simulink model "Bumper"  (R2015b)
settings: Solver=VariableStepAuto  StartTime=0.0  StopTime=10.0  RelTol=1e-3
libraries: vexarmcortexlib x5

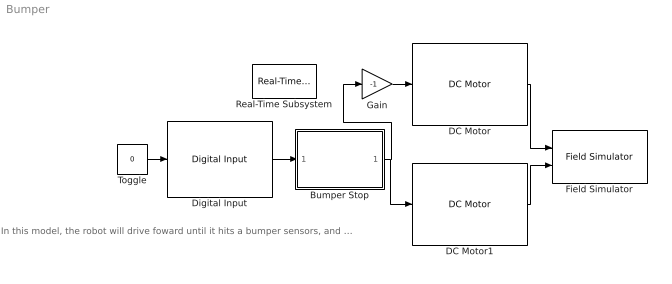
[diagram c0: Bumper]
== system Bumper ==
  note: In this model, the robot will drive foward until it hits a bumper sensors, and then will stop.
  Bumper Stop : Stateflow chart  TreatAsAtomicUnit=on
  DC Motor : vexarmcortexlib/DC Motor  motor=3  scaleFactor=1/13.5  SimulationOut=on
  DC Motor1 : vexarmcortexlib/DC Motor  motor=7  scaleFactor=1/13.5  SimulationOut=on
  Digital Input : vexarmcortexlib/Digital Input  inChan=1  SimulationIn=on
  Field Simulator : vexarmcortexlib/Utilities/Field Simulator  radius=2.5  space=10  range=200
  Gain : Gain  Gain=-1
  Real-Time Subsystem : vexarmcortexlib/Utilities/Real-Time Subsystem  x=1
  Toggle : Constant  Value=0
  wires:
  DC Motor/1 -> Field Simulator/1
  DC Motor1/1 -> Field Simulator/2
  Gain/1 -> DC Motor/1
  Digital Input/1 -> Bumper Stop/1(bumper)
  Bumper Stop/1(speed) -> DC Motor1/1, Gain/1
  Toggle/1 -> Digital Input/1

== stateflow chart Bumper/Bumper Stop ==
  state Drive_Forward
    during:
    speed = 100;
  state Stop
    during:
    speed = 0;
  (default) -> Drive_Forward : {speed = 0;}
  Drive_Forward -> Stop : [bumper == 0]
  data: bumper input; speed output
